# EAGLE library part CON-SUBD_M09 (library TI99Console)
SUB-D
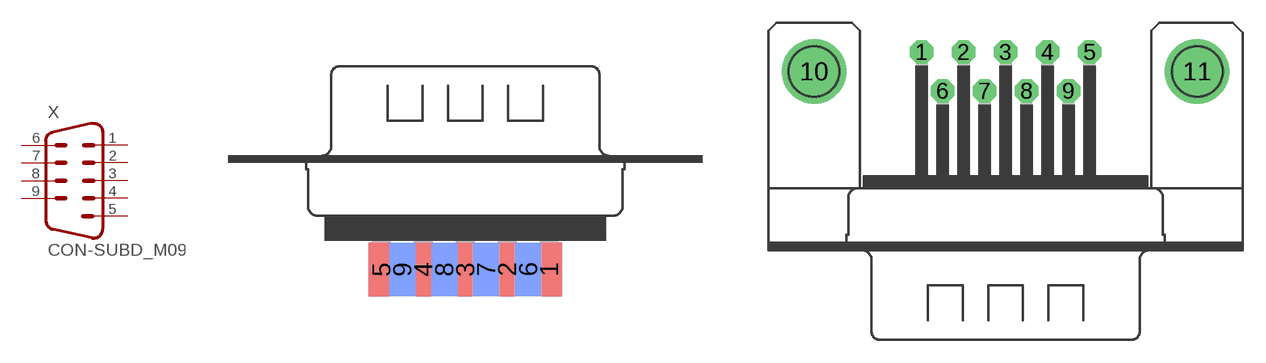
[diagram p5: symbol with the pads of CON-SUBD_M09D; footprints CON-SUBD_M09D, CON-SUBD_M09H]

Designator prefix X

## CON-SUBD_M09D  [CON-SUBD_M09D]
1  1  pas
2  2  pas
3  3  pas
4  4  pas
5  5  pas
6  6  pas
7  7  pas
8  8  pas
9  9  pas

## CON-SUBD_M09H  [CON-SUBD_M09H]
Pads as for CON-SUBD_M09D

## CON-SUBD_M09HP  [CON-SUBD_M09HP]
Pads as for CON-SUBD_M09D

## CON-SUBD_M09V  [CON-SUBD_M09V]
Pads as for CON-SUBD_M09D

## CON-SUBD_M09VB  [CON-SUBD_M09VB]
Pads as for CON-SUBD_M09D

## CON-SUBD_M09VP  [CON-SUBD_M09VP]
Pads as for CON-SUBD_M09D

## Footprint CON-SUBD_M09D (pad centres in mm)
SUB-D
smd 1.7 x 3.5: 1 5.486,-6.045; 2 2.743,-6.045; 3 0,-6.045; 4 -2.743,-6.045; 5 -5.486,-6.045
smd 1.7 x 3.5 bottom: 6 4.115,-6.045; 7 1.372,-6.045; 8 -1.372,-6.045; 9 -4.115,-6.045

## Footprint CON-SUBD_M09H (pad centres in mm)
SUB-D
drill 1.016 octagon: 1 -5.486,1.27; 2 -2.743,1.27; 3 0,1.27; 4 2.743,1.27; 5 5.486,1.27; 6 -4.115,-1.27; 7 -1.372,-1.27; 8 1.372,-1.27; 9 4.115,-1.27
drill 3.2: 10 -12.522,0; 11 12.522,0

## Footprint CON-SUBD_M09HP (pad centres in mm)
SUB-D
drill 1.016 octagon: 1 -5.486,1.27; 2 -2.743,1.27; 3 0,1.27; 4 2.743,1.27; 5 5.486,1.27; 6 -4.115,-1.27; 7 -1.372,-1.27; 8 1.372,-1.27; 9 4.115,-1.27
drill 3.302 pad 5.08: G1 -12.522,0; G2 12.522,0

## Footprint CON-SUBD_M09V (pad centres in mm)
SUB-D
drill 1.016 octagon: 1 -5.486,1.422; 2 -2.743,1.422; 3 0,1.422; 4 2.743,1.422; 5 5.486,1.422; 6 -4.115,-1.422; 7 -1.372,-1.422; 8 1.372,-1.422; 9 4.115,-1.422
hole 3.302 at -12.522,0
hole 3.302 at 12.522,0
